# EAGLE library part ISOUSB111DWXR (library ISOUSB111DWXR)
USB Interface IC Low emissions, full and low speed isolated USB repeater 16-SSOP -40 to 125 Source: Datasheet
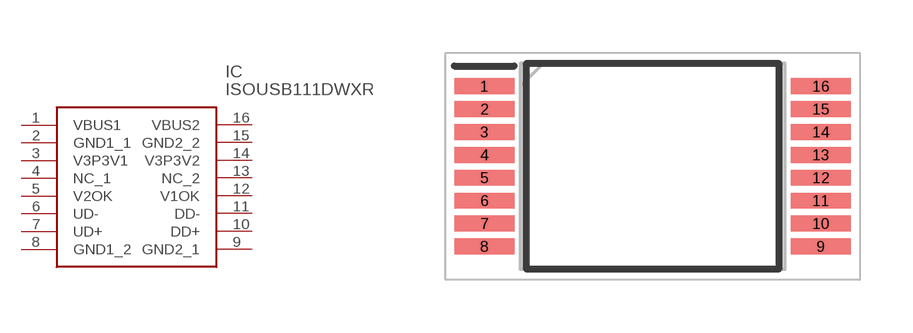
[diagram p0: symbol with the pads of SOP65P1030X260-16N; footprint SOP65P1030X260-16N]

Designator prefix IC

## ISOUSB111DWXR (Description: USB Interface IC Low emissions, full and low speed isolated USB repeater 16-SSOP -40 to 125; Height: 2.6mm; Manufacturer_Name: Texas Instruments; Manufacturer_Part_Number: ISOUSB111DWXR; Mouser_Part_Number: 595-ISOUSB111DWXR; Mouser_Price-Stock: https://www.mouser.co.uk/ProductDetail/Texas-Instruments/ISOUSB111DWXR?qs=Y0Uzf4wQF3msEozH7EwD3g%3D%3D)  [SOP65P1030X260-16N]
1  VBUS1
2  GND1_1
3  V3P3V1
4  NC_1
5  V2OK
6  UD-
7  UD+
8  GND1_2
9  GND2_1
10  DD+
11  DD-
12  V1OK
13  NC_2
14  V3P3V2
15  GND2_2
16  VBUS2

## Footprint SOP65P1030X260-16N (pad centres in mm)
ISOUSB111DWXR
smd 1.7 x 0.45: 1 -4.775,2.275; 2 -4.775,1.625; 3 -4.775,0.975; 4 -4.775,0.325; 5 -4.775,-0.325; 6 -4.775,-0.975; 7 -4.775,-1.625; 8 -4.775,-2.275; 9 4.775,-2.275; 10 4.775,-1.625; 11 4.775,-0.975; 12 4.775,-0.325; 13 4.775,0.325; 14 4.775,0.975; 15 4.775,1.625; 16 4.775,2.275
